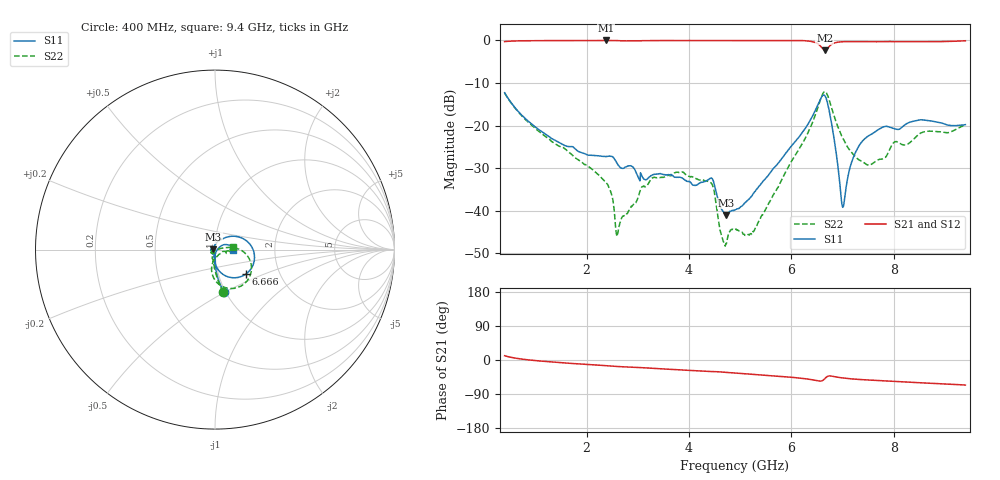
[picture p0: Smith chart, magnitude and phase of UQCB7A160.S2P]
!  Part Number  UQCB7A160	Mounting Orientation: Vertical
!  Description: RF capacitors
!  Application: Coupling, Bypass, Tuning, DC Block
!  Filters, Matching
# GHZ S DB R 50
! Freq  |S11|  S11 Ph  |S21|  S21 Ph  |S12|  S12 Ph  |S22|  S22 Ph
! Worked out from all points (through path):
!   801 points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, 400 MHz to 9.4 GHz, reference 50 ohm
!   highest |S21| = 0.00 dB at 2.38 GHz (marker M1); lowest = -2.3 dB at 6.655 GHz (marker M2)
!   group delay of S21, straight-line fit = 21.6 ps
!   lowest |S11| = -41.0 dB at 4.731 GHz (marker M3), VSWR 1.02, Z = 49.1 + j0.231 ohm
!   |S11| at or under -10 dB: start of sweep to end of sweep
!   |S22| runs from -48.3 to -12.0 dB; largest |S21 - S12| = 0.0012
!   S11 on the Smith chart (normalised r, x): 400 MHz: 0.98, -0.50; 6.666 GHz: 1.34, -0.39; 9.4 GHz: 1.23, -0.01
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0.4  -12.28 -78.3  -0.27 11.3  -0.27 11.3  -12.31 -79.0
0.996  -20.29 -89.2  -0.05 -1.5  -0.06 -1.5  -20.62 -93.1
1.908  -26.38 -91.4  -0.03 -10.8  -0.03 -10.8  -28.58 -115.3
2.38  -27.26 -89.9  0.00 -14.8  -0.01 -14.9  -33.36 -150.5
2.493  -27.22 -94.8  -0.01 -16.0  -0.01 -16.0  -36.29 -176.2
2.605  -29.00 -99.6  -0.04 -17.2  -0.05 -17.2  -45.43 -155.5
3.089  -32.01 -116.9  -0.06 -20.2  -0.06 -20.2  -34.34 -108.2
3.404  -31.33 -109.4  -0.03 -22.8  -0.03 -22.8  -32.20 -119.1
4.416  -32.38 -168.0  -0.03 -30.4  -0.03 -30.4  -33.33 -172.7
4.641  -39.71 159.0  -0.01 -32.0  -0.01 -32.0  -46.08 -171.7
4.731  -40.98 164.7  -0.01 -32.9  -0.01 -32.9  -47.74 -126.4
4.9  -39.77 155.5  -0.01 -34.4  -0.01 -34.4  -44.40 -107.8
5.249  -36.08 118.3  -0.01 -37.9  -0.01 -37.9  -44.85 -48.6
6.408  -17.90 35.8  -0.28 -52.1  -0.28 -52.1  -19.44 5.8
6.655  -12.98 -33.4  -2.32 -49.1  -2.32 -49.1  -12.01 -49.1
6.666  -13.19 -39.1  -2.30 -47.5  -2.30 -47.5  -12.05 -54.1
6.813  -21.38 -87.6  -0.74 -43.1  -0.74 -43.1  -16.85 -95.4
7.004  -39.18 -33.3  -0.30 -47.4  -0.30 -47.4  -22.92 -99.0
7.161  -29.20 30.4  -0.26 -49.7  -0.25 -49.7  -26.07 -88.4
7.33  -24.56 28.1  -0.27 -51.4  -0.27 -51.4  -28.09 -72.4
7.904  -20.28 4.1  -0.26 -55.7  -0.26 -55.7  -26.08 -10.9
9.4  -19.77 -1.6  -0.07 -66.2  -0.07 -66.2  -19.74 6.6
